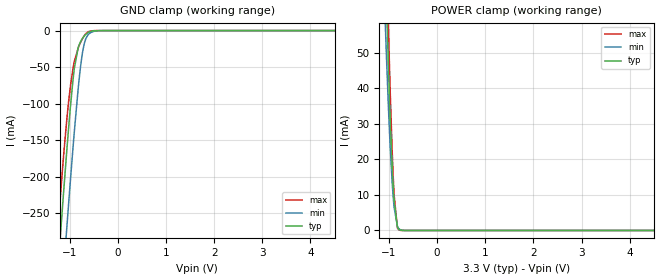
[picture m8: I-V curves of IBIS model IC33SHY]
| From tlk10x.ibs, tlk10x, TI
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|   Model
[Model]   IC33SHY
Model_type   Input
Vinl = 0.99
Vinh = 2.31
|   typ   min   max
C_comp   1.468pF   1.430pF   1.519pF
[Voltage Range]   3.3   3   3.6
[Temperature Range]   25   125   -40
[Power Clamp Reference]   3.3   3   3.6
[GND Clamp Reference]   -0   -0   -0
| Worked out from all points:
|   GND clamp passes 1 mA (typ) near -0.56 V on its own axis
|   POWER clamp passes 1 mA (typ) near -0.82 V on its own axis
[GND Clamp]
|   Voltage   I(typ)   I(min)   I(max)
-3.3V     -2.326A    -2.431A    -2.267A
-1.251V   -331.2mA   -441.1mA   -274.2mA
-1.142V   -233mA     -341.3mA   -181.8mA
-1.063V   -164.7mA   -270.5mA   -122.4mA
-993.3mV  -109.4mA   -210.3mA   -79.85mA
-924mV    -62.17mA   -152.8mA   -48.47mA
-825mV    -23.15mA   -79.06mA   -23.83mA
-765.6mV  -13.88mA   -43.78mA   -14.71mA
-716.1mV  -8.837mA   -23.09mA   -8.683mA
-597.3mV  -1.939mA   -4.277mA   -1.186mA
-270.6mV  -1.831uA   -18.3uA    -237.6nA
6.59V     0A         0A         0A
[POWER Clamp]
|   Voltage   I(typ)   I(min)   I(max)
-3.3V     1.527A     1.443A     1.596A
-1.082V   79.31mA    60.57mA    96.18mA
-1.063V   69.42mA    52.79mA    84.76mA
-1.053V   64.64mA    49.06mA    79.17mA
-1.013V   46.77mA    35.23mA    57.82mA
-1.003V   42.65mA    32.05mA    52.8mA
-973.5mV  31.18mA    23.26mA    38.67mA
-933.9mV  18.2mA     13.54mA    22.49mA
-894.3mV  8.483mA    6.621mA    10.1mA
-825mV    1.027mA    1.217mA    784.3uA
-785.4mV  229.6uA    397.4uA    113.8uA
6.59V     0A         0A         0A
